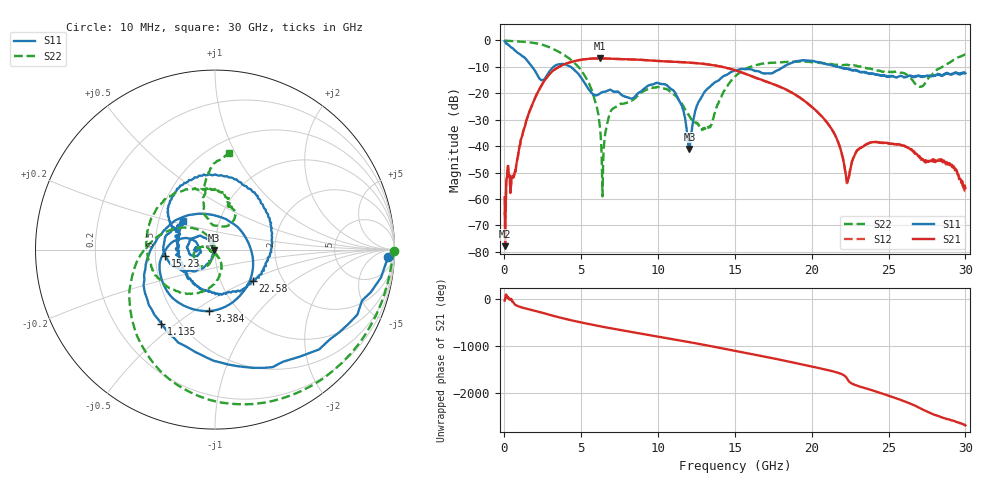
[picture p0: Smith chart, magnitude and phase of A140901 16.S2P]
!  2-Port S-parameters saved by WinCal
! VAR MeasName=S-Parameters (CALIBRATED_DATA) read from VNA (N5244A)
! VAR MeasDate=11/3/2014 9:27:59 AM
! VAR NAME=A140901 16
! VAR FILENAME=A140901 16.S2P
! VAR DATE=11/3/2014 9:27:59 AM
! VAR PHYS_PORTS=1,2
# Hz S RI R 50
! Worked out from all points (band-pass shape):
!   801 points, 10 MHz to 30 GHz, reference 50 ohm
!   highest |S21| = -6.79 dB at 6.233 GHz (marker M1); lowest = -77.9 dB at 47.49 MHz (marker M2)
!   |S21| within 3 dB of the highest: 3.619 GHz to 14 GHz (10.38 GHz wide, 118 % of centre)
!   lowest |S11| = -41.1 dB at 12.04 GHz (marker M3), VSWR 1.02, Z = 49.2 - j0.324 ohm
!   |S11| at or under -10 dB: 1.796 GHz to 3.194 GHz (1.397 GHz wide, 56 % of centre); 4.316 GHz to 18.16 GHz (13.85 GHz wide, 123 % of centre); 21.67 GHz to end of sweep
!   |S22| runs from -59.0 to 0.0 dB; largest |S21 - S12| = 0.004
!   S11 on the Smith chart (normalised r, x): 10 MHz: 24, -28; 1.135 GHz: 0.40, -0.44; 3.384 GHz: 0.75, -0.58; 15.23 GHz: 0.57, -0.04; 22.58 GHz: 1.42, -0.53; 30 GHz: 0.67, +0.23
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1e7  0.9649 -0.0396  0.000749 -0.000754  0.000239 0.000515  0.9985 -0.00869
4.74875e7  0.9248 -0.1555  0.000128 5.94e-06  0.000338 0.000279  0.9938 -0.0373
4.973375e8  0.3206 -0.6549  0.00116 -0.00241  0.00121 -0.00238  0.9219 -0.3094
1.134625e9  -0.2985 -0.4127  -0.0149 0.0026  -0.0149 0.00248  0.7067 -0.6316
2.146788e9  -0.0929 0.2  0.00561 0.1014  0.00556 0.1012  0.1333 -0.8614
3.383875e9  -0.031 -0.3419  0.2716 -0.1176  0.2714 -0.1171  -0.4379 -0.471
5.033325e9  -0.1782 0.0624  -0.3651 -0.2326  -0.365 -0.2327  -0.2361 0.1124
5.895538e9  -0.0903 0.0108  -0.4123 0.1938  -0.4125 0.1934  -0.0283 0.0666
6.232925e9  -0.0997 -0.00661  -0.3145 0.3325  -0.3144 0.3318  -0.00427 0.0202
8.294738e9  -0.0783 -0.0145  0.4274 0.0946  0.4265 0.0943  -0.0281 -0.0676
1.001916e10  -0.1554 0.0185  0.0358 -0.4075  0.0354 -0.4066  -0.1159 -0.0631
1.118128e10  -0.0643 0.0664  -0.3414 -0.1944  -0.3421 -0.1941  -0.0857 0.0123
1.204349e10  -0.0082 -0.00329  -0.3565 0.1332  -0.356 0.1329  -0.0359 0.00646
1.335555e10  -0.0766 -0.1058  0.0605 0.3417  0.0622 0.3419  0.000753 -0.0238
1.5005e10  -0.2582 -0.0662  0.2483 -0.1133  0.2457 -0.1158  -0.0194 -0.2061
1.522992e10  -0.2768 -0.0344  0.202 -0.1637  0.2006 -0.1636  -0.0566 -0.2281
2.002832e10  0.0969 0.4  0.0541 0.00352  0.0543 0.00377  -0.2384 0.3029
2.227758e10  0.2614 -0.1207  -0.00111 0.00193  -0.000924 0.00176  -0.0396 0.343
2.257748e10  0.2108 -0.1722  0.00439 0.000987  0.00444 0.000686  -0.0123 0.3334
2.501416e10  -0.1651 -0.1195  -0.0035 0.0107  -0.00338 0.0108  0.0774 0.2449
2.711346e10  -0.2022 0.0106  -0.00567 -0.00176  -0.00528 -0.00154  0.00392 0.1332
3e10  -0.1767 0.1609  -0.00148 -0.000618  -0.00134 -0.000405  0.0761 0.538
